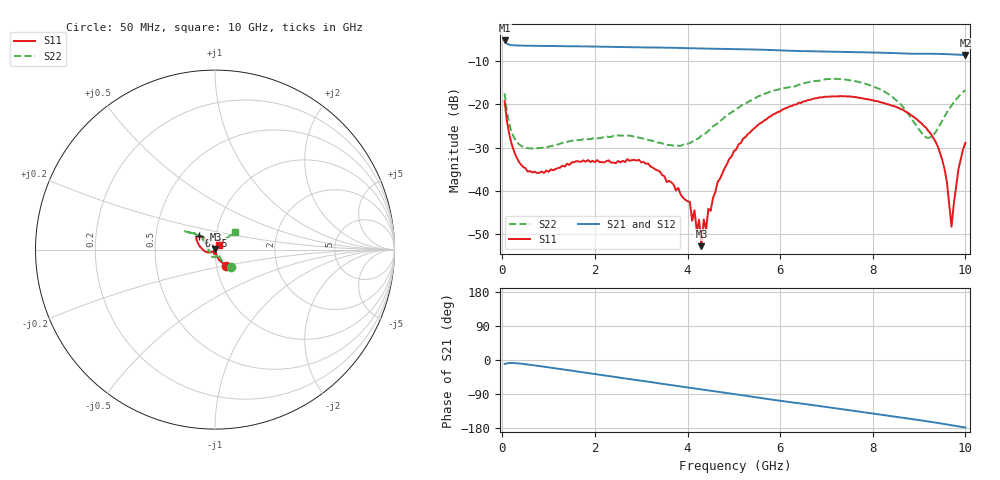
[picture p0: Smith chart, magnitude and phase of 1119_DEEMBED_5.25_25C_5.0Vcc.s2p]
!Hittite Microwave Corp.
!Digital Attenuator/PhaseShifter Rev 1.4.0
!Filename: C:\DATA\DATA\1119_DEEMBED_5.25_25C_5.0Vcc.s2p
!VNA ID: Agilent Technologies,N5224A,MY51441122,A.10.45.03
!Device type:
!2 Port Calibration.
!Temp(C): 25
!Lot Number:
!Serial Number:
!Operator:
!Misc:
!Attenuator:  5.250
# GHZ S DB R 50.0
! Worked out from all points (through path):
!   200 points, 50 MHz to 10 GHz, reference 50 ohm
!   highest |S21| = -5.21 dB at 50 MHz (marker M1); lowest = -8.6 dB at 10 GHz (marker M2)
!   group delay of S21, straight-line fit = 48.3 ps
!   lowest |S11| = -52.8 dB at 4.3 GHz (marker M3), VSWR 1.00, Z = 50.2 + j0.0662 ohm
!   |S11| at or under -10 dB: start of sweep to end of sweep
!   |S22| runs from -30.2 to -14.1 dB; largest |S21 - S12| = 0.0016
!   S11 on the Smith chart (normalised r, x): 50 MHz: 1.11, -0.20; 6.75 GHz: 0.83, +0.13; 10 GHz: 1.05, +0.06
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0.05  -19.24 -55.4  -5.21 -10.4  -5.21 -10.4  -17.45 -47.5
0.2  -29.17 -74.7  -6.29 -7.8  -6.29 -7.8  -26.38 -58.1
0.55  -35.59 -78.3  -6.43 -11.8  -6.43 -11.8  -30.16 -53.5
1.75  -32.97 -101.5  -6.58 -32.7  -6.59 -32.7  -28.09 -80.4
3.4  -35.51 -89.6  -6.85 -61.7  -6.86 -61.8  -28.88 -137.5
4.05  -42.57 -56.1  -7.00 -73.2  -7.01 -73.3  -28.99 -177.7
4.2  -49.39 -23.6  -7.05 -76.0  -7.06 -76.0  -28.06 170.7
4.25  -46.70 -6.5  -7.06 -76.8  -7.07 -76.9  -27.80 168.7
4.3  -52.83 16.8  -7.07 -77.6  -7.08 -77.7  -27.22 164.6
4.35  -46.66 37.7  -7.08 -78.5  -7.09 -78.5  -26.96 160.8
4.4  -49.07 52.1  -7.08 -79.4  -7.10 -79.5  -26.66 159.0
4.65  -37.99 99.8  -7.13 -83.7  -7.16 -83.7  -24.38 147.6
5.05  -30.47 118.0  -7.21 -90.7  -7.23 -90.7  -21.10 139.5
6.7  -18.77 138.9  -7.72 -119.0  -7.73 -119.0  -14.68 147.3
6.75  -18.60 138.8  -7.73 -119.8  -7.75 -119.9  -14.60 147.5
8.35  -20.04 160.2  -8.10 -147.6  -8.10 -147.6  -17.70 138.6
9.15  -25.40 -167.2  -8.28 -161.3  -8.30 -161.3  -27.63 108.6
9.35  -28.54 -154.6  -8.30 -165.1  -8.32 -165.1  -26.55 73.7
9.55  -35.02 -136.4  -8.36 -169.1  -8.37 -169.1  -22.77 50.7
9.7  -48.30 -74.2  -8.42 -172.1  -8.44 -172.1  -20.28 44.0
9.85  -35.03 38.3  -8.50 -175.2  -8.51 -175.2  -18.23 42.2
10  -28.89 48.1  -8.60 -178.2  -8.61 -178.2  -16.74 41.5
